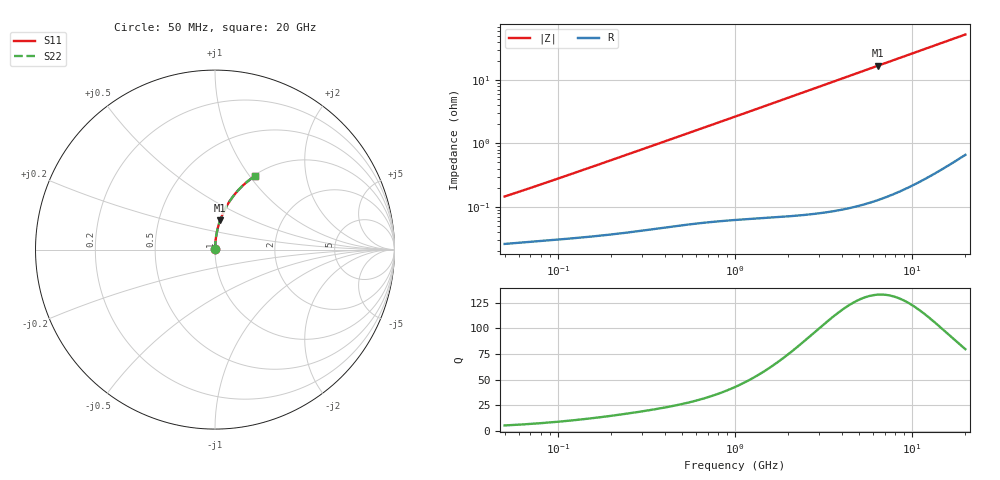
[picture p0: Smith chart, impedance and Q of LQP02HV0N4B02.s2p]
!Murata Part Number: LQP02HV0N4B02
!These Parameters are Measured in Series Mode Connection
!  o--[Z]--o
!Port1  Port2
!  o-------o
!Freq. Start=50[MHz] Stop=20[GHz], 401[Steps]
# Hz S RI R 50
!Freq.(Hz) S11(Real) S11(Imag) S21(Real) S21(Imag) S12(Real) S12(Imag) S22(Real) S22(Imag)
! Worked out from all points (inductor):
!   401 points, 50 MHz to 20 GHz, reference 50 ohm
!   read as one part in series: L = 448 pH near 51.52 MHz
!   highest Q = 133 at 6.407 GHz (marker M1), where L = 419 pH
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5e7  0.00026 0.00143  0.9997 -0.00143  0.9997 -0.00143  0.00026 0.00143
5.152053e7  0.000262 0.00147  0.9997 -0.00147  0.9997 -0.00147  0.000262 0.00147
6.951576e7  0.000282 0.00195  0.9997 -0.00195  0.9997 -0.00195  0.000282 0.00195
1.364002e8  0.00034 0.00373  0.9997 -0.00373  0.9997 -0.00373  0.00034 0.00373
3.721004e8  0.000554 0.00998  0.9994 -0.00998  0.9994 -0.00998  0.000554 0.00998
6.380365e8  0.000838 0.017  0.9992 -0.017  0.9992 -0.017  0.000838 0.017
1e9  0.00132 0.0264  0.9987 -0.0264  0.9987 -0.0264  0.00132 0.0264
1.714689e9  0.00272 0.0451  0.9973 -0.0451  0.9973 -0.0451  0.00272 0.0451
2.728004e9  0.0059 0.0714  0.9941 -0.0714  0.9941 -0.0714  0.0059 0.0714
3.415248e9  0.00885 0.0891  0.9912 -0.0891  0.9912 -0.0891  0.00885 0.0891
4.275624e9  0.0134 0.1111  0.9866 -0.1111  0.9866 -0.1111  0.0134 0.1111
5.273168e9  0.02 0.136  0.98 -0.136  0.98 -0.136  0.02 0.136
6.406762e9  0.0289 0.1637  0.9711 -0.1637  0.9711 -0.1637  0.0289 0.1637
7.442007e9  0.0383 0.1883  0.9617 -0.1883  0.9617 -0.1883  0.0383 0.1883
9.892087e9  0.0653 0.2431  0.9347 -0.2431  0.9347 -0.2431  0.0653 0.2431
1.115139e10  0.0814 0.2692  0.9186 -0.2692  0.9186 -0.2692  0.0814 0.2692
1.257102e10  0.101 0.2968  0.899 -0.2968  0.899 -0.2968  0.101 0.2968
1.417136e10  0.1247 0.3256  0.8753 -0.3256  0.8753 -0.3256  0.1247 0.3256
1.573793e10  0.1493 0.3512  0.8507 -0.3512  0.8507 -0.3512  0.1493 0.3512
1.747767e10  0.1777 0.3766  0.8223 -0.3766  0.8223 -0.3766  0.1777 0.3766
1.940974e10  0.2101 0.4013  0.7899 -0.4013  0.7899 -0.4013  0.2101 0.4013
2e10  0.2202 0.4081  0.7798 -0.4081  0.7798 -0.4081  0.2202 0.4081
